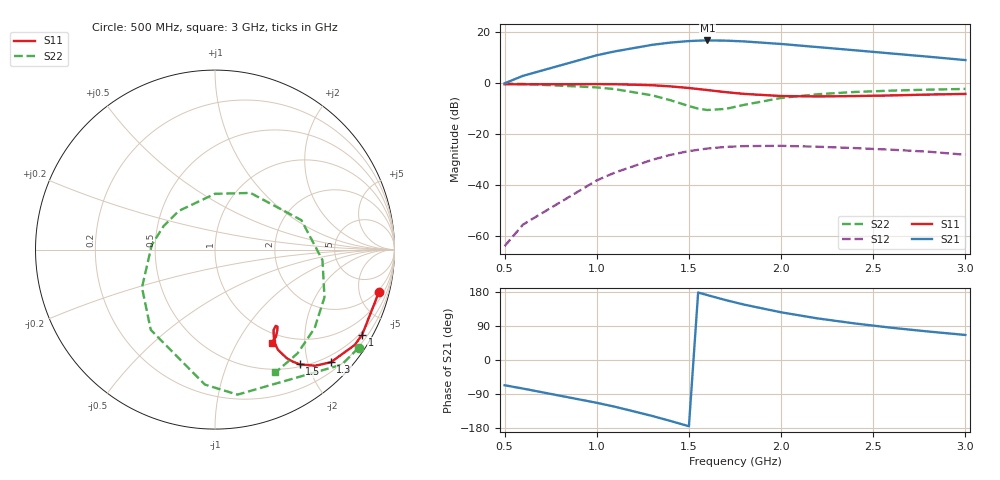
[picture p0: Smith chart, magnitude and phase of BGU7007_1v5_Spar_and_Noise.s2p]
! BGU7007, Vcc=1.50 V, Icc=4.5935 mA
# MHz S MA R 50
!  Freq-MHz  S11-mag  S11-arg  S21-mag  S21-arg  S12-mag  S12-arg  S22-mag  S22-arg
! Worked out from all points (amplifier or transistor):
!   17 points, 500 MHz to 3 GHz, reference 50 ohm
!   highest |S21| = 16.6 dB at 1.6 GHz (marker M1)
!   |S21| within 3 dB of that: 1.199 GHz to 2.265 GHz (1.066 GHz wide, 61.6 % of centre)
!   unconditionally stable (mu >= 1): start of sweep to 1.078 GHz; 1.998 GHz to end of sweep
!   at 1 GHz: K = 1.07, MAG = 22.8 dB, |S12| = -38.1 dB
!   at 1.6 GHz: K = 0.92, MSG = 21.1 dB, |S12| = -25.6 dB
!   at 3 GHz: K = 1.53, MAG = 14.2 dB, |S12| = -28.1 dB
!   lowest NFmin = 0.71 dB at 1.1 GHz
!   S11 on the Smith chart (normalised r, x): 500 MHz: 1.79, -7.49; 1 GHz: 0.40, -3.69; 1.3 GHz: 0.36, -2.41; 1.5 GHz: 0.54, -1.86; 3 GHz: 0.85, -1.41
500  0.9422 -14.4  0.9827 -66.7  0.0006461 -85.5  0.9697 -34.4
600  0.9396 -17.0  1.376 -75.4  0.001709 -103.6  0.9536 -42.2
1000  0.9469 -30.0  3.47 -113.0  0.01247 -146.2  0.8176 -81.2
1100  0.9429 -34.3  4.141 -123.5  0.01782 -157.5  0.7543 -94.3
1300  0.9003 -44.2  5.537 -147.6  0.03136 178.5  0.5727 -128.7
1400  0.8551 -49.2  6.138 -160.9  0.03929 164.9  0.4585 -152.5
1500  0.7952 -53.5  6.566 -174.8  0.04651 151.1  0.3531 175.5
1550  0.7595 -55.2  6.69 178.2  0.04932 144.2  0.3147 155.4
1600  0.7251 -56.5  6.75 171.2  0.0522 137.6  0.2954 133.1
1700  0.6595 -57.9  6.693 158.0  0.05618 124.2  0.3108 90.0
1800  0.6098 -57.3  6.464 146.1  0.05825 112.8  0.3725 58.0
2000  0.5543 -54.0  5.763 125.9  0.05891 93.6  0.5085 18.8
2200  0.5431 -51.4  5.004 109.7  0.05661 79.0  0.6015 -5.6
2400  0.5534 -51.0  4.341 96.5  0.05331 67.7  0.6652 -23.5
2600  0.5693 -52.4  3.755 85.0  0.04949 58.5  0.7069 -38.3
2800  0.5922 -55.0  3.249 75.1  0.0453 50.9  0.7387 -51.5
3000  0.609 -58.6  2.79 66.1  0.03946 44.8  0.7628 -63.8
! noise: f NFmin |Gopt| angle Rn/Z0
500  0.7902  0.5201  15.32  0.2919
600  0.7322  0.5189  15.64  0.2656
1100  0.7083  0.4244  25.78  0.2224
1400  0.7479  0.4369  30.1  0.2383
1550  0.7159  0.4259  32.37  0.2181
1600  0.7112  0.4211  34.24  0.218
1800  0.7261  0.4261  37.32  0.2134
2200  0.824  0.3984  46.02  0.2131
2600  0.9671  0.3734  56.13  0.2092
3000  1.119  0.4042  65.04  0.2349
